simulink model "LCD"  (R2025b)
settings: Solver=FixedStepAuto  StartTime=0.0  StopTime=10  RelTol=1e-3  EnableMultiTasking=on

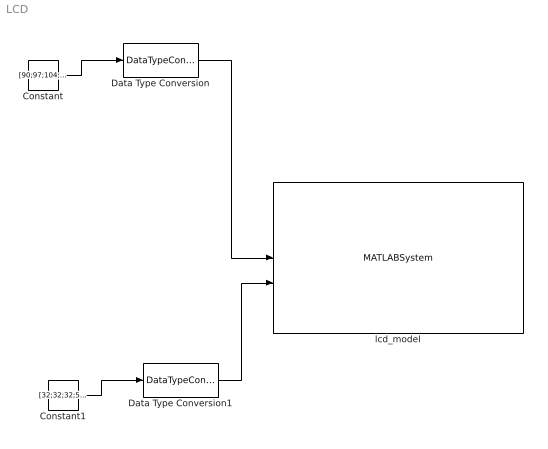
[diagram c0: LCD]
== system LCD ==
  Constant : Constant  Value=[90;97;104;108;101;110;99;111;100;101;58;32;49;47;52;32]
  Constant1 : Constant  Value=[32;32;32;51;32;32;53;32;32;49;32;32;52;32;32;32]
  Data Type Conversion : DataTypeConversion  OutDataTypeStr=uint8
  Data Type Conversion1 : DataTypeConversion  OutDataTypeStr=uint8
  lcd_model : MATLABSystem  System=lcd  SampleTime=-1
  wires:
  Constant/1 -> Data Type Conversion/1
  Constant1/1 -> Data Type Conversion1/1
  Data Type Conversion1/1 -> lcd_model/2
  Data Type Conversion/1 -> lcd_model/1
